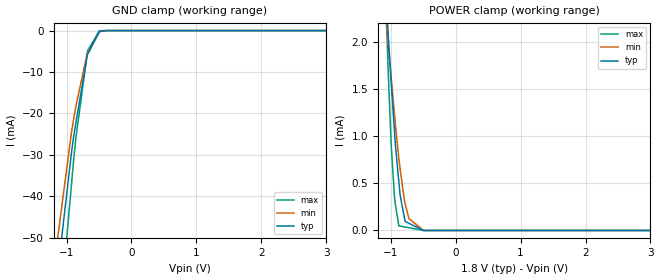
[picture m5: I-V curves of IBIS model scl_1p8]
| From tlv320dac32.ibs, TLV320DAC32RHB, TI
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|   scl_1p8 Model
[Model]   scl_1p8
Model_type   Input
Vinl = 0.54
Vinh = 1.26
|   typ   min   max
|   (nom PVT)   (fast PVT)   (slow PVT)
|C_comp from frequency sweep method (F=0.4MHz)
|Average
|C_comp   3.650e-12   3.632e-12   3.670e-12
|C_comp from LC tank measurement(L=1nH)
|Average
|Resonant Frequency(Hz)   4.630e+09   4.640e+09   4.620e+09
C_comp   1.183e-12   1.178e-12   1.188e-12
[Model spec]
|subparameter   typ   min   max
Vinl   0.54   0.486   0.594
Vinh   1.26   1.134   1.386
| Where nom  PVT is Nominal Process, 1.8V, 45C
|   Fast PVT is Strong Process,  1.98V, -40C
|   Slow PVT is Weak Process,   1.62V, 105C
[Voltage Range]   1.8   1.62   1.98
|Ambient Temperature   25   85   -40
|Junction Temperature
[Temperature Range]   45   105   -40
[Power Clamp Reference]   1.8   1.62   1.98
[GND Clamp Reference]   0   0   0
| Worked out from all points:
|   GND clamp passes 1 mA (typ) near -0.52 V on its own axis
|   POWER clamp passes 1 mA (typ) near -0.94 V on its own axis
[GND Clamp]
|   Voltage   I(typ)   I(min)   I(max)
-1.8V     -227.9mA   -129.7mA   -345.2mA
-1.137V   -58.37mA   -50.11mA   -75.07mA
-923.4mV  -29.45mA   -24.53mA   -37.1mA
-891mV    -25.62mA   -21.49mA   -31.32mA
-855.4mV  -22.29mA   -18.29mA   -25.85mA
-690.1mV  -6.845mA   -6.13mA    -6.624mA
-680.4mV  -5.936mA   -5.596mA   -5.493mA
-675.2mV  -5.776mA   -5.449mA   -4.886mA
-495mV    -240.3uA   -380.2uA   -65.71uA
-426.1mV  -44.37uA   -83.05uA   -6.449uA
-307.8mV  -1.264uA   -4.601uA   -85.81nA
3.6V      0A         0A         0A
[POWER Clamp]
|   Voltage   I(typ)   I(min)   I(max)
-1.8V     11.87mA    8.619mA    19.35mA
-1.085V   2.649mA    2.361mA    2.616mA
-1.039V   2.086mA    1.979mA    1.704mA
-990mV    1.542mA    1.604mA    881.4uA
-938.5mV  1.023mA    1.21mA     323.2uA
-923.4mV  874.4uA    1.094mA    257.8uA
-875.2mV  522uA      770.1uA    49.36uA
-855mV    374.8uA    656.9uA    46.74uA
-777.6mV  96.52uA    281.9uA    36.69uA
-719.3mV  76.6uA     126.4uA    29.12uA
-494.1mV  11.68nA    505.4nA    0A
3.6V      0A         0A         0A
